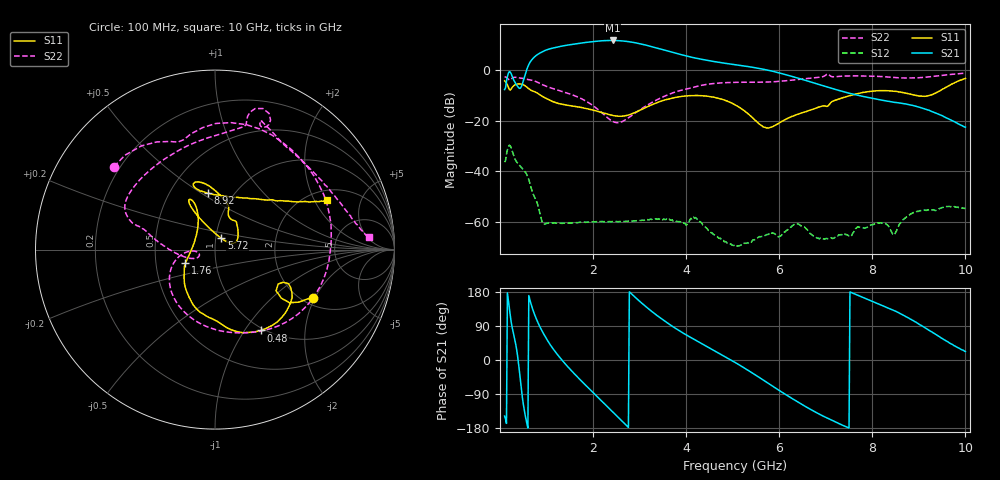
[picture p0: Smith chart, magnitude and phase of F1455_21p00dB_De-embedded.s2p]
! Integrated Device Technology
! Corporate Headquarters
! 6024 Silver Creek Valley Road
! San Jose, CA 95138  USA
! Phone:  1-408-284-8200
! Toll Free:  1-800-223-1366
! Webpage:  http://www.idt.com/
! Timing and RF Division
! 515 Groton Road, Suite 102
! Westford, MA 01886-6024
! Device:  F1455
! Description: 6-bit 0.5 dB Transmit Variable Gain Amplifier
! Frequency:  1400.0 -  2300.00 MHz
! Package:  6x6 mm Thin QFN Plastic Package: 28 pin
! State:  42
! Atten State:  21.0 dB
! Voltage:  +5.00 Volts
! Current:  217.625 mA
! Data:  The device was measured on a the F1455 evaluation board which has
!  individual transmission lines to the RF pins.  Data was collected
!  using a calibrated network analyzer.  The evaluation board was
!  de-embedded using a TRL calibration technique.
!  The reference plane is the edge of the package pin.
!  Pin  1 = CSb
!  Pin  2 = DATA
!  Pin  3 = CLK
!  Pin  4 = RSET
!  Pin  5 = GND
!  Pin  6 = RFIN  = Port 1
!  Pin  7 = GND
!  Pin  8 = NC
!  Pin  9 = NC
!  Pin 10 = NC
!  Pin 11 = NC
!  Pin 12 = NC
!  Pin 13 = NC
!  Pin 14 = /STBY
!  Pin 15 = GND
!  Pin 16 = RFOUT  = Port 2
!  Pin 17 = GND
!  Pin 18 = NC
!  Pin 19 = NC
!  Pin 20 = NC
!  Pin 21 = GND
!  Pin 22 = NC
!  Pin 23 = GND
!  Pin 24 = NC
!  Pin 25 = NC
!  Pin 26 = NC
!  Pin 27 = GND
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# GHz S dB R 50
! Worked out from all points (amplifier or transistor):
!   496 points, 100 MHz to 10 GHz, reference 50 ohm
!   highest |S21| = 11.6 dB at 2.42 GHz (marker M1)
!   |S21| within 3 dB of that: 1.137 GHz to 3.38 GHz (2.242 GHz wide, 99.3 % of centre)
!   unconditionally stable (mu >= 1): start of sweep to end of sweep
!   at 1.74 GHz: K = 132.52, MAG = 11.1 dB, |S12| = -60.0 dB
!   at 5.06 GHz: K = 744.99, MAG = 3.9 dB, |S12| = -69.3 dB
!   at 10 GHz: K = 488.20, MAG = -13.9 dB, |S12| = -54.5 dB
!   S11 on the Smith chart (normalised r, x): 100 MHz: 2.26, -1.93; 480 MHz: 0.97, -1.20; 1.76 GHz: 0.71, -0.11; 5.72 GHz: 1.06, +0.14; 8.92 GHz: 0.76, +0.53; 10 GHz: 2.46, +2.51
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0.1  -4.32 -26.2  -7.74 -148.1  -36.35 47.3  -2.75 140.7
0.18  -6.78 -36.2  -1.35 159.3  -30.24 -7.2  -3.70 112.7
0.26  -6.93 -24.8  -2.41 87.3  -31.80 -77.0  -3.31 95.9
0.38  -5.55 -42.0  -6.50 9.6  -36.77 -117.4  -3.03 57.9
0.48  -5.69 -60.2  -5.62 -96.9  -38.84 -148.8  -3.32 31.7
0.68  -8.13 -90.3  3.90 142.9  -47.09 139.4  -4.05 -14.9
0.82  -9.35 -108.7  6.22 97.5  -53.67 111.7  -4.96 -45.9
0.96  -10.93 -123.4  7.59 64.4  -60.77 126.1  -6.19 -71.2
1.34  -13.54 -144.6  9.41 -1.4  -60.48 101.1  -8.49 -121.0
1.76  -14.83 -155.7  10.62 -56.6  -59.99 70.1  -11.43 -156.2
2.1  -16.34 -165.6  11.34 -97.9  -59.89 52.3  -15.49 -174.1
2.42  -17.90 175.6  11.61 -136.9  -59.68 40.6  -20.26 -170.8
2.82  -17.38 139.0  10.98 175.2  -59.55 29.4  -18.12 -157.0
3.1  -15.08 122.2  9.92 144.4  -59.25 23.4  -14.65 -169.1
3.4  -12.72 115.1  8.50 115.2  -58.70 11.8  -11.55 178.4
4.1  -10.13 116.1  5.07 59.4  -58.51 -5.1  -7.14 163.1
5.06  -13.80 116.8  2.05 -7.0  -69.29 -12.0  -4.89 148.2
5.72  -22.82 61.0  0.04 -57.9  -65.02 4.9  -4.79 121.1
6.7  -15.66 39.2  -4.88 -132.2  -64.89 -127.9  -3.21 78.5
8.36  -8.22 107.8  -12.45 135.9  -61.91 90.2  -2.82 62.6
8.92  -9.97 97.0  -14.23 100.8  -55.96 111.7  -3.15 40.1
10  -3.35 23.8  -22.55 22.2  -54.53 34.2  -1.28 4.6
